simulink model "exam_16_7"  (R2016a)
settings: Solver=VariableStepAuto  StartTime=0.0  StopTime=10.0  RelTol=1e-3

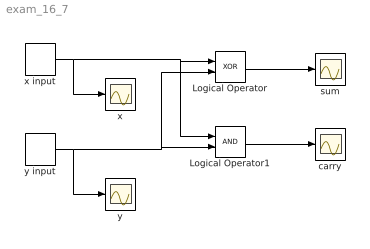
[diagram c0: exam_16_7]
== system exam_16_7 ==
  Logical Operator : Logic  Operator=XOR  AllPortsSameDT=off  OutDataTypeStr=boolean
  Logical Operator1 : Logic  AllPortsSameDT=off  OutDataTypeStr=boolean
  carry : Scope
  sum : Scope
  x : Scope
  x input : DiscretePulseGenerator  PulseType=Time based  Period=4  PulseWidth=50  PhaseDelay=2
  y : Scope
  y input : DiscretePulseGenerator  PulseType=Time based  Period=8  PulseWidth=50  PhaseDelay=4
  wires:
  x input/1 -> x/1, Logical Operator1/1, Logical Operator/1
  y input/1 -> y/1, Logical Operator1/2, Logical Operator/2
  Logical Operator/1 -> sum/1
  Logical Operator1/1 -> carry/1
